(* Logix 5000 AddOnInstructionDefinition export AlicatUpdateInput; software revision 20.04 *)

TYPE AlicatIoData :
STRUCT
   Status : DINT;   // Device Status Flags
   T_OVER : BOOL;   // Temperature Overflow
   T_UNDR : BOOL;   // Temperature Underflow
   V_OVER : BOOL;   // Volumetric Overflow
   V_UNDR : BOOL;   // Volumetric Underflow
   M_OVER : BOOL;   // Mass Overflow
   M_UNDR : BOOL;   // Mass Underflow
   P_OVER : BOOL;   // Pressure Overflow
   TOT_OVER : BOOL;   // Totalizer Overflow
   HLD : BOOL;   // PID Loop in Hold
   ADC : BOOL;   // ADC Error
   EXH : BOOL;   // PID Exhaust
   OPL : BOOL;   // Over Pressure Limit
   TMF : BOOL;   // Flow Overflow During Totalize
   Pressure : REAL;
   Temperature : REAL;
   VolFlow : REAL;
   MassFlow : REAL;
   ActualSetpoint : REAL;
   ValveDrivePct : REAL;
   Totalizer : REAL;
   RequestedSetpoint : REAL;
   GasIndex : INT;
   Config : SINT;
   PRESS : BOOL;   // Pressure Reading Valid
   TEMP : BOOL;   // Temperature Reading Valid
   VFLOW : BOOL;   // Volumetric Flow Reading Valid
   MFLOW : BOOL;   // Mass Flow Reading Valid
   SP : BOOL;   // Setpoint Reading Valid
   VDRIVE : BOOL;   // Valve Drive Percentage Reading Valid
   TOTAL : BOOL;   // Totalizer Reading Valid
END_STRUCT
END_TYPE

ADD_ON_INSTRUCTION AlicatUpdateInput   (* revision 1.0, vendor Alicat Scientific, Inc *)
// Updates AlicatIoData UDT from device input data array.
// Help:
// This AOI copies input data from an Alicat IO device into a UDT which allows accessing data readings as REAL values. It also decodes the device status word into status flags. Since RSLogix performs device IO asynchronously, it is recommended to copy the input data into a SINT array with the CPS instruction before calling this AOI.
// Before calling, set the flags in IoData.Config to match the configuration of your device. See the Alicat operating bulletin for more information.
VAR_IN_OUT
   InputArray : SINT[6]; {required}   // Array of SINTs from device input data.
   IoData : AlicatIoData; {required}   // AlicatIoData UDT to update.
END_VAR
VAR
   InputSize : DINT; {access None}
   InputOffset : DINT; {access None}
END_VAR

ROUTINE Logic   (* ladder *)
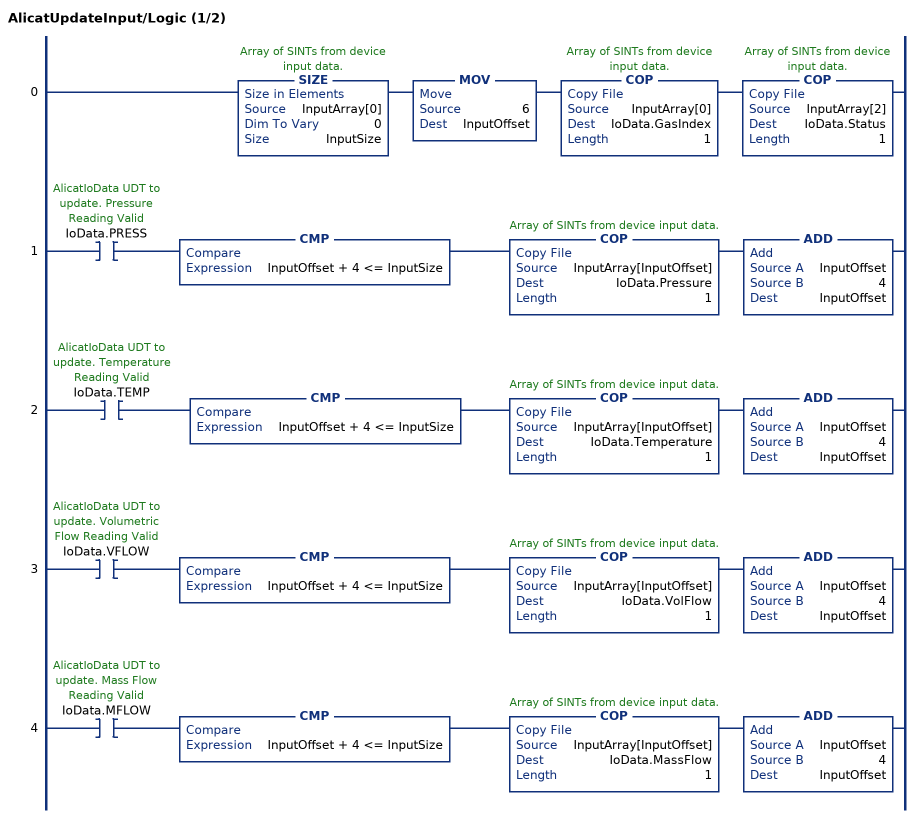
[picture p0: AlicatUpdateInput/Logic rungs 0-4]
   0: SIZE(InputArray[0],0,InputSize)MOV(6,InputOffset)COP(InputArray[0],IoData.GasIndex,1)COP(InputArray[2],IoData.Status,1);
   1: XIC(IoData.PRESS)CMP(InputOffset + 4 <= InputSize)COP(InputArray[InputOffset],IoData.Pressure,1)ADD(InputOffset,4,InputOffset);
   2: XIC(IoData.TEMP)CMP(InputOffset + 4 <= InputSize)COP(InputArray[InputOffset],IoData.Temperature,1)ADD(InputOffset,4,InputOffset);
   3: XIC(IoData.VFLOW)CMP(InputOffset + 4 <= InputSize)COP(InputArray[InputOffset],IoData.VolFlow,1)ADD(InputOffset,4,InputOffset);
   4: XIC(IoData.MFLOW)CMP(InputOffset + 4 <= InputSize)COP(InputArray[InputOffset],IoData.MassFlow,1)ADD(InputOffset,4,InputOffset);
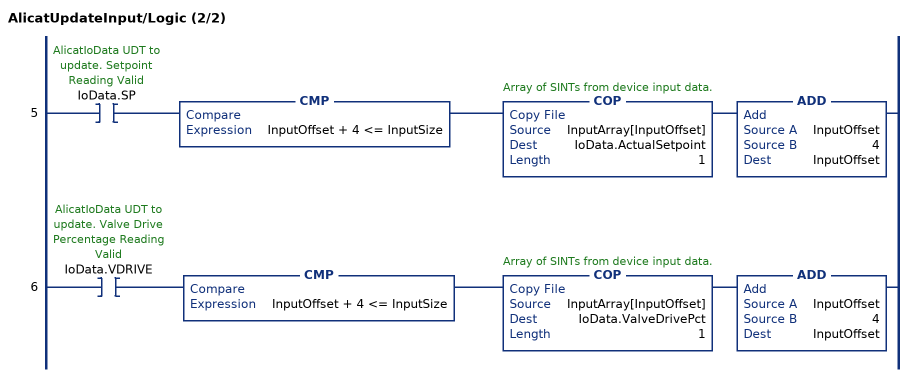
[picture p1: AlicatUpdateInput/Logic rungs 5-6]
   5: XIC(IoData.SP)CMP(InputOffset + 4 <= InputSize)COP(InputArray[InputOffset],IoData.ActualSetpoint,1)ADD(InputOffset,4,InputOffset);
   6: XIC(IoData.VDRIVE)CMP(InputOffset + 4 <= InputSize)COP(InputArray[InputOffset],IoData.ValveDrivePct,1)ADD(InputOffset,4,InputOffset);
END_ROUTINE
END_ADD_ON_INSTRUCTION
